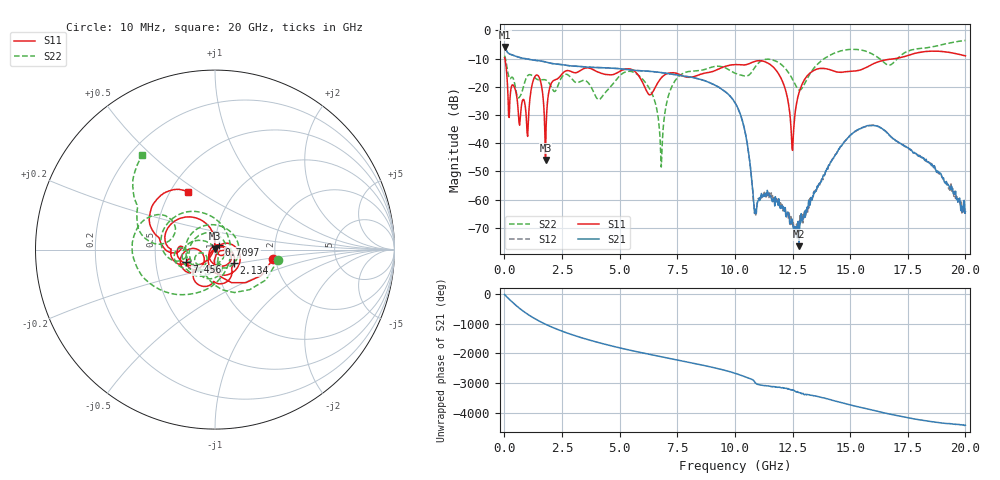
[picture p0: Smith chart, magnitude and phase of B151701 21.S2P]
!  2-Port S-parameters saved by WinCal
! VAR MeasName=S-Parameters (CALIBRATED_DATA) read from VNA (N5244A)
! VAR MeasDate=2015-12-24 19:10:36
! VAR NAME=B151701 21
! VAR FILENAME=B151701 21.S2P
! VAR DATE=2015-12-24 19:10:36
! VAR PHYS_PORTS=1,3
# Hz S DB R 50
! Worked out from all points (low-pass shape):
!   801 points, 10 MHz to 20 GHz, reference 50 ohm
!   highest |S21| = -5.88 dB at 10 MHz (marker M1); lowest = -76.5 dB at 12.78 GHz (marker M2)
!   |S21| within 3 dB of the highest: start of sweep to 390.1 MHz
!   lowest |S11| = -46.0 dB at 1.784 GHz (marker M3), VSWR 1.01, Z = 50 + j0.502 ohm
!   |S11| at or under -10 dB: 18.73 MHz to 16.95 GHz (16.93 GHz wide, 200 % of centre)
!   |S22| runs from -48.4 to -3.6 dB; largest |S21 - S12| = 0.0035
!   S11 on the Smith chart (normalised r, x): 10 MHz: 1.94, -0.23; 709.6 MHz: 1.05, +0.06; 2.134 GHz: 1.22, -0.19; 7.456 GHz: 0.72, -0.10; 20 GHz: 0.61, +0.45
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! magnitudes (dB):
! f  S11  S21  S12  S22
! 10 MHz  -9.7  -5.9  -5.9  -9.0
! 709.6 MHz  -29.0  -9.7  -9.7  -22.9
! 1.01 GHz  -37.6  -10.2  -10.2  -16.1
! 1.409 GHz  -15.8  -10.7  -10.7  -17.3
! 1.784 GHz  -46.0  -11.2  -11.2  -17.6
! 2.134 GHz  -17.8  -11.8  -11.8  -21.4
! 3.358 GHz  -13.9  -12.8  -12.8  -17.9
! 4.108 GHz  -14.9  -13.2  -13.2  -24.5
! 5.657 GHz  -14.5  -14.2  -14.2  -15.0
! 6.682 GHz  -18.2  -14.8  -14.8  -31.5
! 6.832 GHz  -16.6  -15.0  -15.0  -43.3
! 7.456 GHz  -15.2  -15.7  -15.7  -17.3
! 10.01 GHz  -12.1  -25.6  -25.6  -15.2
! 10.45 GHz  -12.2  -36.5  -36.4  -16.2
! 10.88 GHz  -11.0  -64.1  -64.0  -13.0
! 11.98 GHz  -16.6  -63.1  -61.1  -11.9
! 12.48 GHz  -41.7  -66.8  -67.0  -17.0
! 12.78 GHz  -22.2  -76.5  -67.6  -21.1
! 13.35 GHz  -14.5  -60.1  -59.3  -14.2
! 15.13 GHz  -14.4  -36.3  -36.5  -6.7
! 16.68 GHz  -10.3  -36.9  -36.9  -12.3
! 20 GHz  -9.0  -64.2  -65.2  -3.6
